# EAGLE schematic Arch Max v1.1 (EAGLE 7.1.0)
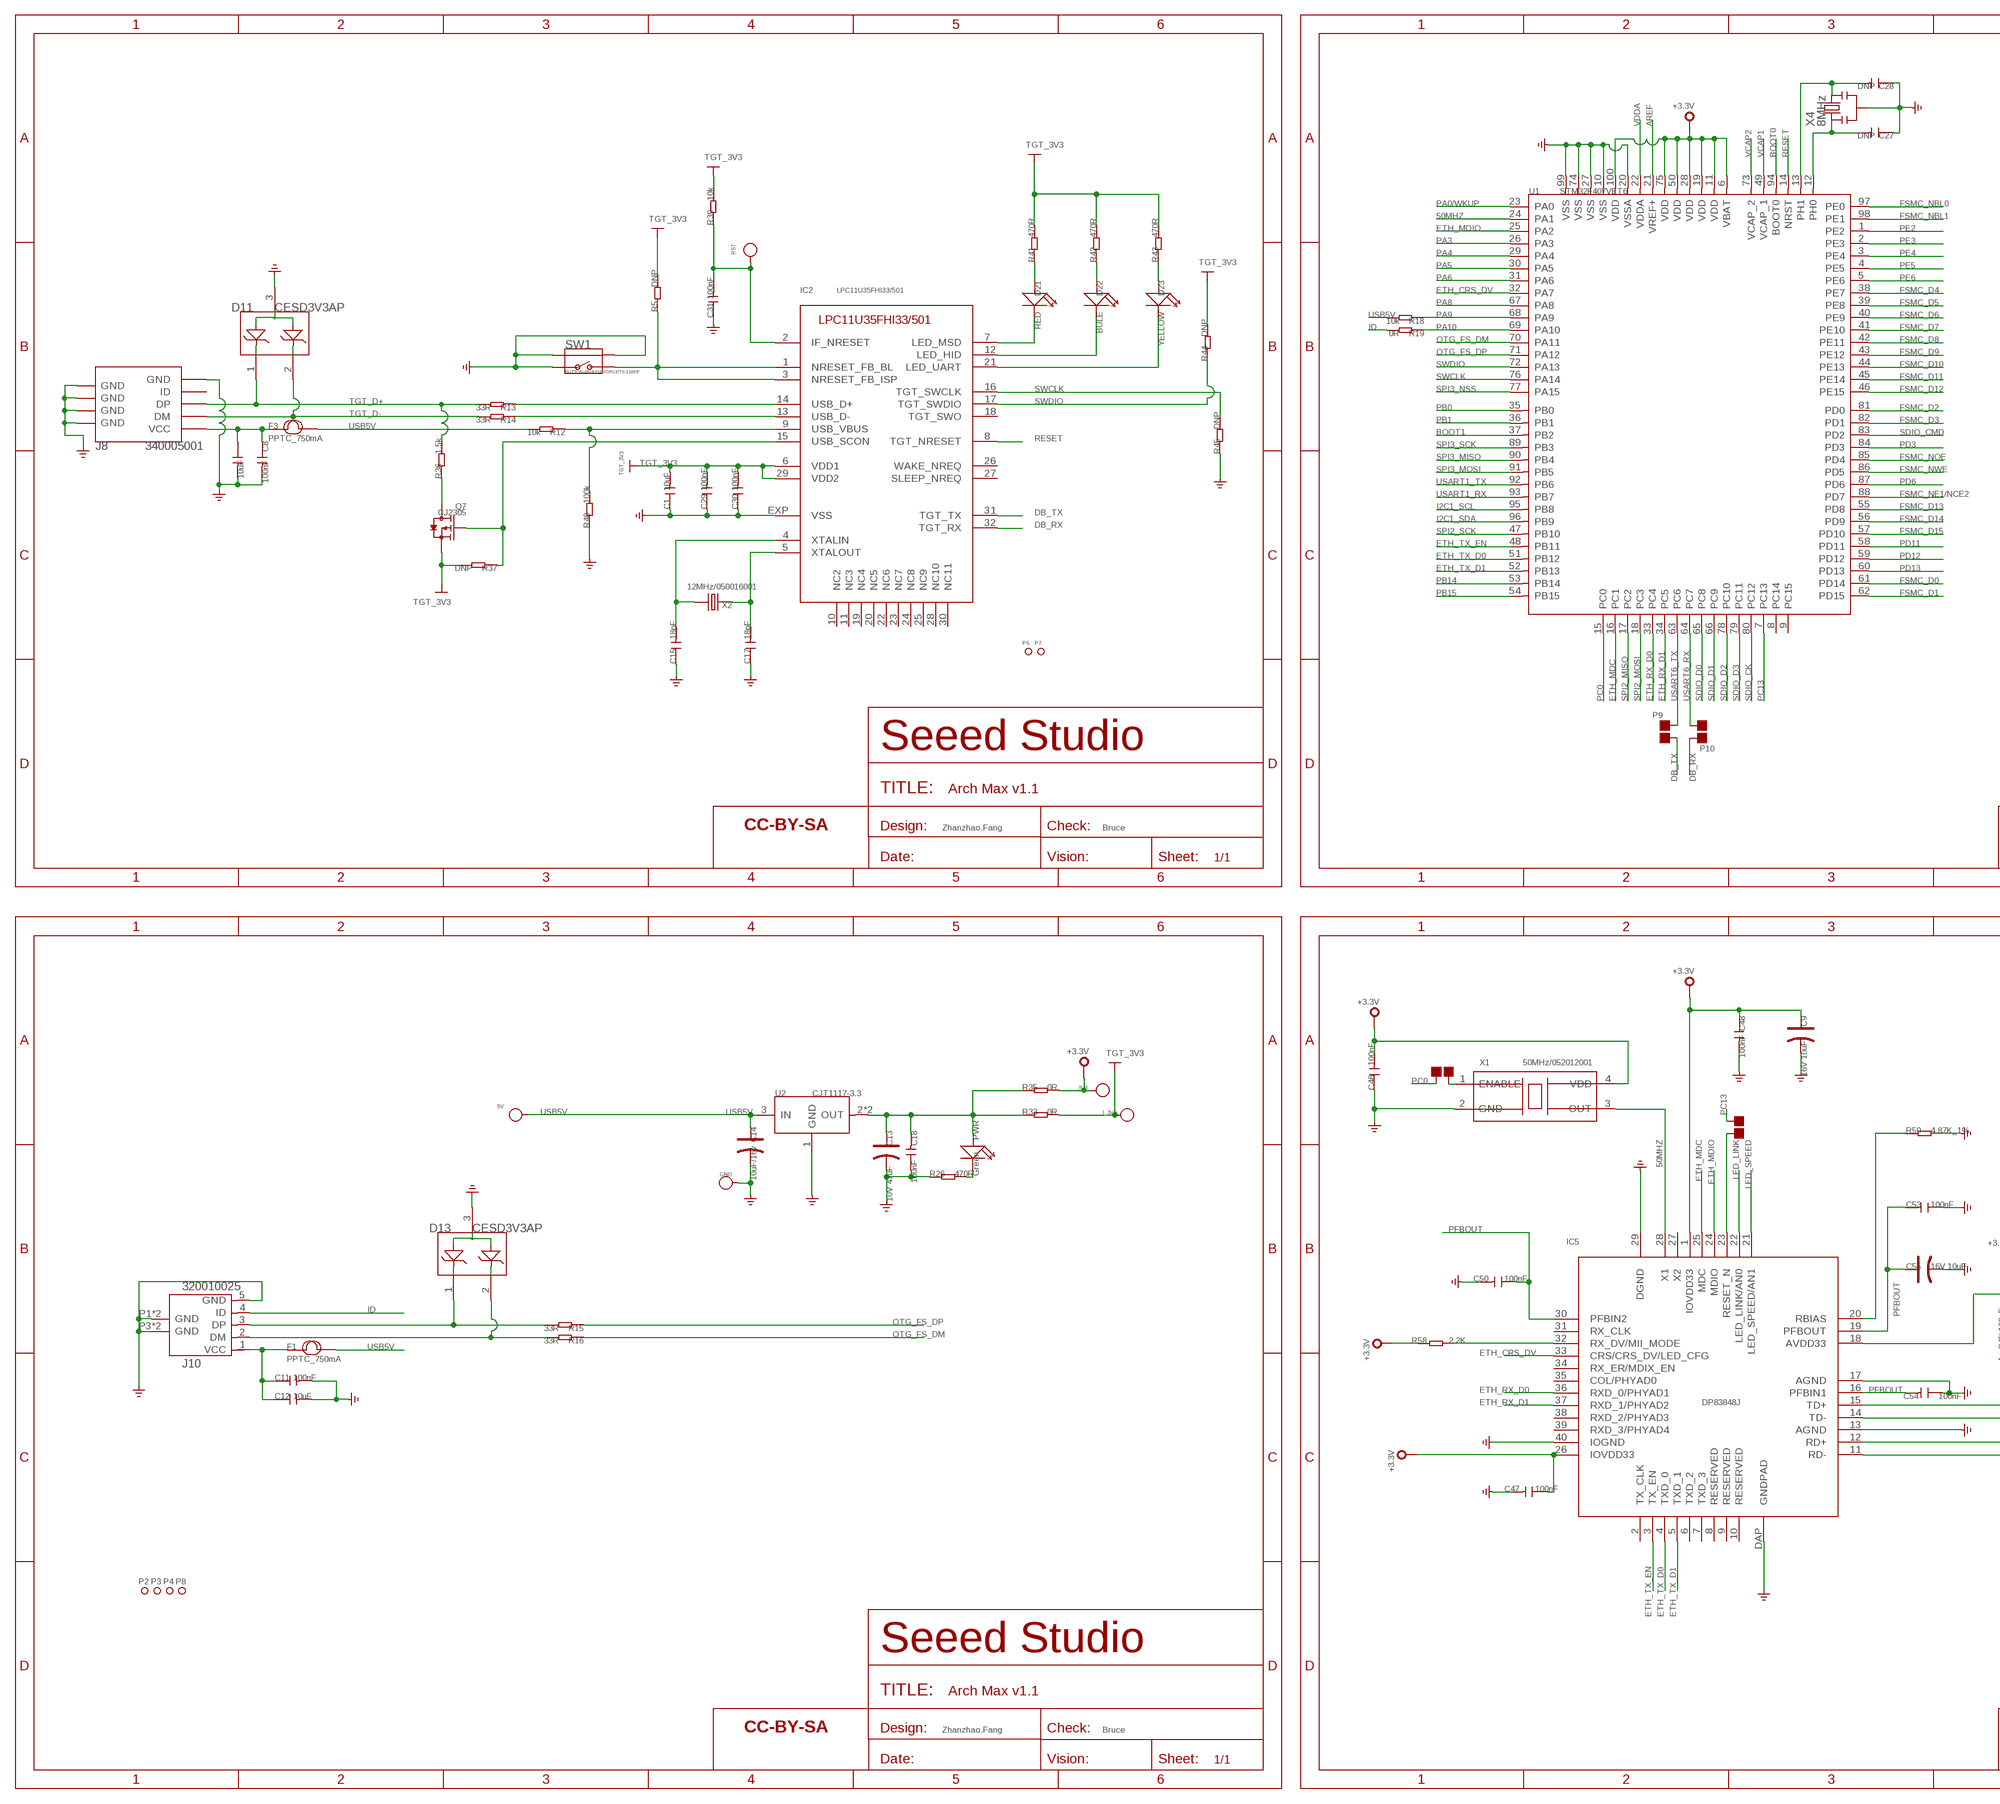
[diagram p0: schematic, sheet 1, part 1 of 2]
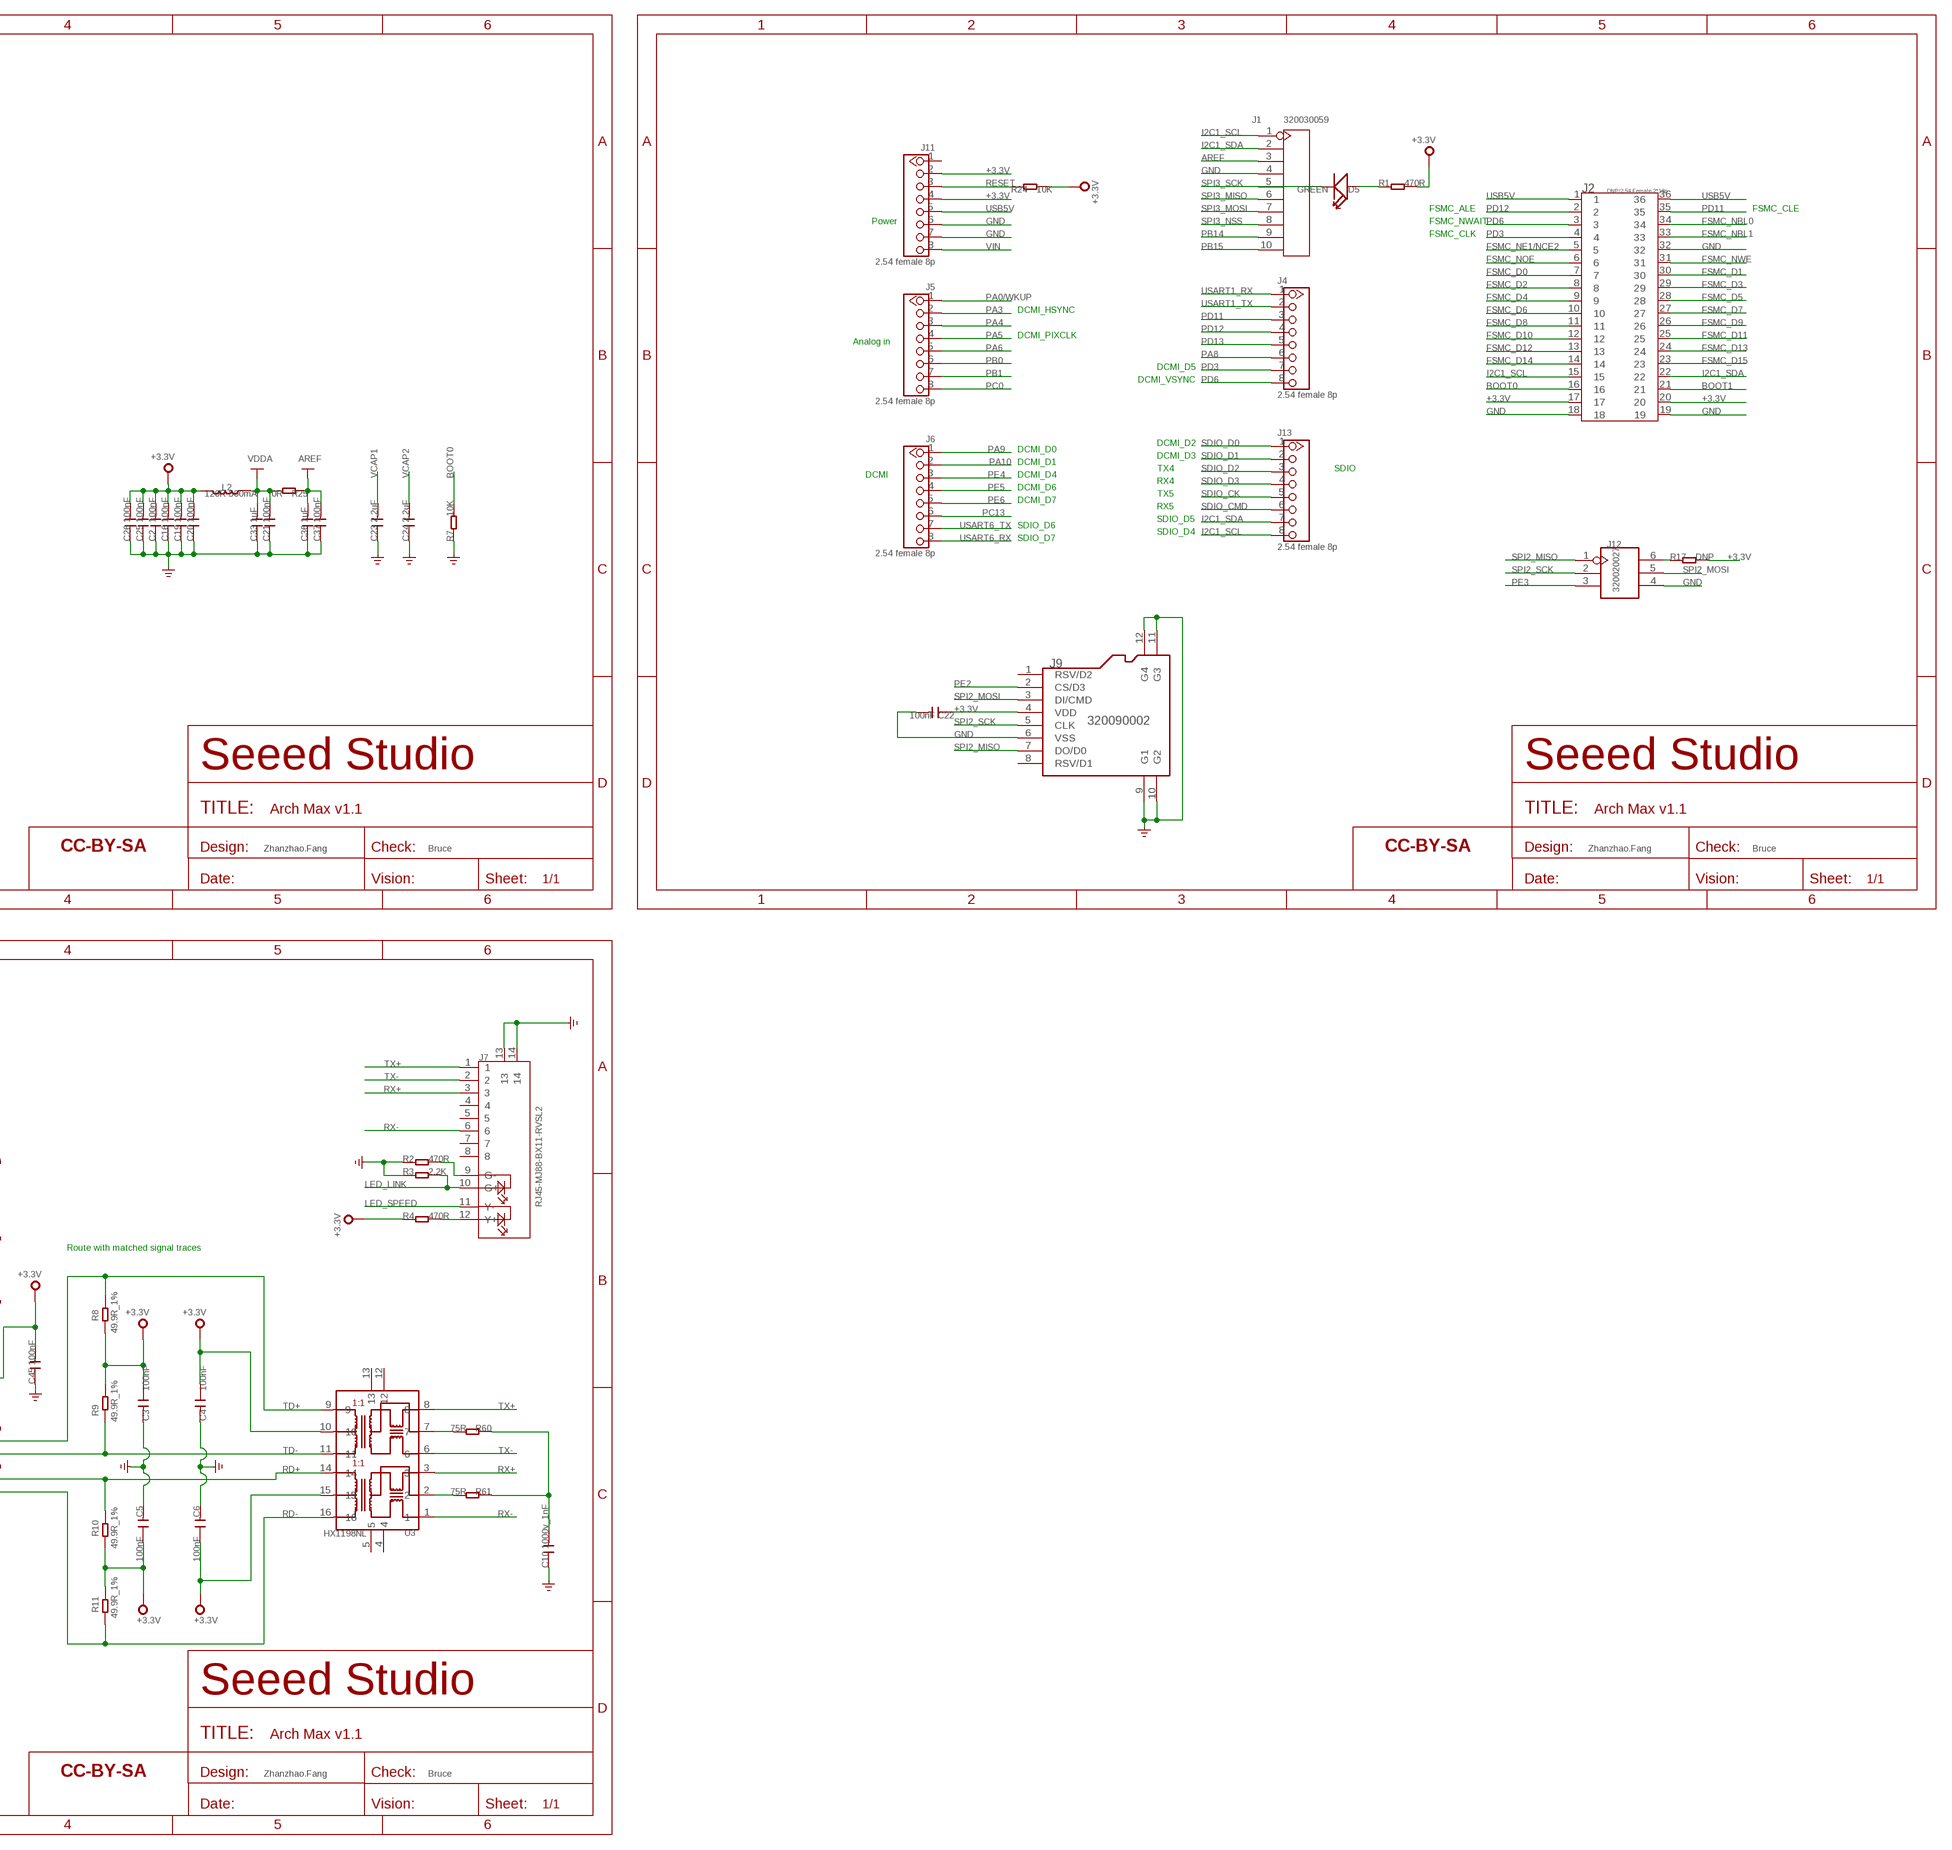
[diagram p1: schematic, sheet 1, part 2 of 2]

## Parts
3V3  NC  PAD-TEST-POINT'4545'  [TP_4545]
5V  NC  PAD-TEST-POINT'4545'  [TP_4545]
C1  10uF  C-0805  [C0805]
C2  100nF  C-0603  [C0603]
C3  100nF  C-0603  [C0603]
C4  100nF  C-0603  [C0603]
C5  100nF  C-0603  [C0603]
C6  100nF  C-0603  [C0603]
C7  10uF  C-0805  [C0805]
C8  100nF  C-0603  [C0603]
C9  16V 10uF  CAP-AVX-A  [AVX-A]
C10  1000v_1nF  C-1206  [C1206]
C11  100nF  C-0603  [C0603]
C12  10uF  C-0805  [C0805]
C13  10V 47uF  CAP-AVX-B  [AVX-B]
C14  10uF/16v  CAP-AVX-A  [AVX-A]
C15  18pF  C-0603  [C0603]
C16  100nF  C-0603  [C0603]
C17  18pF  C-0603  [C0603]
C18  100nF  C-0603  [C0603]
C19  100nF  C-0603  [C0603]
C20  100nF  C-0603  [C0603]
C21  100nF  C-0603  [C0603]
C22  100nF  C-0603  [C0603]
C23  2.2uF  C-0603  [C0603]
C24  2.2uF  C-0603  [C0603]
C25  100nF  C-0603  [C0603]
C26  100nF  C-0603  [C0603]
C27  DNP  C-0603  [C0603]
C28  DNP  C-0603  [C0603]
C29  100nF  C-0603  [C0603]
C30  100nF  C-0603  [C0603]
C31  100nF  C-0603  [C0603]
C33  1uF  C-0603  [C0603]
C36  1uF  C-0603  [C0603]
C37  100nF  C-0603  [C0603]
C45  100nF  C-0603  [C0603]
C46  100nF  C-0603  [C0603]
C47  100nF  C-0603  [C0603]
C48  100nF  C-0603  [C0603]
C50  100nF  C-0603  [C0603]
C53  100nF  C-0603  [C0603]
C54  100nF  C-0603  [C0603]
C55  16V 10uF  CAP-AVX-A  [AVX-A]
D5  GREEN  LED'0603'  [LED-0603]
D11  CESD3V3AP  D-ESD-3P  [SOT23]
D13  CESD3V3AP  D-ESD-3P  [SOT23]
D21  RED  LED'0603'  [LED-0603]
D22  BULE  LED'0603'  [LED-0603]
D23  YELLOW  LED'0603'  [LED-0603]
F1  PPTC_750mA  FUSE'1206'  [F1206]
F3  PPTC_750mA  FUSE'1206'  [F1206]
GND  NC  PAD-TEST-POINT'4545'  [TP_4545]
I_3V3  NC  PAD-TEST-POINT'4545'  [TP_4545]
IC2  LPC11U35FHI33/501  MBED-ICS_IF-LPC11U35  [MBED-ICS_HVQFN33]
IC5  DP83848J  [LLP-40]
J1  320030059  HEADER-10P-2.54  [10P-2.54-65/35MIL]
J2  DNP/2.54 Female 2*18p  HEADER-2X18P  [2.54-2X18P]
J4  2.54 female 8p  HEADER-8P2.54  [CK_1X8]
J5  2.54 female 8p  HEADER-8P2.54  [CK_1X8]
J6  2.54 female 8p  HEADER-8P2.54  [CK_1X8]
J7  RJ45-MJ88-BX11-RVSL2  [RJ45-MJ88-BX11-RVSL2]
J8  340005001  USB-MINIUSB-5P-MICRO  [MICRO-USB]
J9  320090002  HOLDER-MICROSD-8P  [8P-SMD]
J10  320010025  USB-MICRO-5P'AB'  [MICRO-USB-5P-AB]
J11  2.54 female 8p  HEADER-8P2.54  [CK_1X8]
J12  320020027  HEADER-2X3P-65/35MIL  [2X3P-2.54-65/35MIL]
J13  2.54 female 8p  HEADER-8P2.54  [CK_1X8]
L2  120R-500mA  L'0603'  [L0603]
P1  NC  PAD-JUMPER-2P  [2P-SMD-1.78X1.27]
P2  NC  PAD-MARK'ANNULAR'  [ROUND-MARK-1.0]
P3  NC  PAD-MARK'ANNULAR'  [ROUND-MARK-1.0]
P4  NC  PAD-MARK'ANNULAR'  [ROUND-MARK-1.0]
P5  NC  PAD-JUMPER-2P  [2P-SMD-1.78X1.27]
P6  NC  PAD-MARK'ANNULAR'  [ROUND-MARK-1.0]
P7  NC  PAD-MARK'ANNULAR'  [ROUND-MARK-1.0]
P8  NC  PAD-MARK'ANNULAR'  [ROUND-MARK-1.0]
P9  NC  PAD-JUMPER-2P  [2P-SMD-1.78X1.27]
P10  NC  PAD-JUMPER-2P  [2P-SMD-1.78X1.27]
PWR  Green  LED'0603'  [LED-0603]
Q7  CJ2305  MOSFET-P'SI2323CDS/SI2305DS<BR>'  [SOT23]
R1  470R  R-0603  [R0603]
R2  470R  R-0603  [R0603]
R3  2.2K  R-0603  [R0603]
R4  470R  R-0603  [R0603]
R5  DNP  R-0603  [R0603]
R7  10K  R-0603  [R0603]
R8  49.9R_1%  R-0603  [R0603]
R9  49.9R_1%  R-0603  [R0603]
R10  49.9R_1%  R-0603  [R0603]
R11  49.9R_1%  R-0603  [R0603]
R12  10k  R-0603  [R0603]
R13  33R  R-0603  [R0603]
R14  33R  R-0603  [R0603]
R15  33R  R-0603  [R0603]
R16  33R  R-0603  [R0603]
R17  DNP  R-0603  [R0603]
R18  10k  R-0603  [R0603]
R19  0R  R-0603  [R0603]
R24  10K  R-0603  [R0603]
R25  0R  R-0603  [R0603]
R26  470R  R-0603  [R0603]
R33  0R  R-0603  [R0603]
R35  0R  R-0603  [R0603]
R36  1.5k  R-0603  [R0603]
R37  DNP  R-0603  [R0603]
R39  10k  R-0603  [R0603]
R40  100k  R-0603  [R0603]
R41  470R  R-0603  [R0603]
R42  470R  R-0603  [R0603]
R43  470R  R-0603  [R0603]
R44  DNP  R-0603  [R0603]
R45  DNP  R-0603  [R0603]
R58  2.2K  R-0603  [R0603]
R59  4.87K_1%  R-0603  [R0603]
R60  75R  R-0603  [R0603]
R61  75R  R-0603  [R0603]
RST  NC  PAD-TEST-POINT'4545'  [TP_4545]
SW1  BUTTON-4P-REINFORCE'TS-1188E'  [4P-SMD-7X3.5X3.5H]
U1  STM32F407VET6  [LQFP100]
U2  CJT1117-3.3  LD1117S  [SOT-223]
U3  HX1198NL  [SOIC16-9.53]
U$1  SEEEDSTUDIO-OPEN-SCH-FRAME  [SEEEDSTUDIO-PCB-FRAME]
U$2  SEEEDSTUDIO-OPEN-SCH-FRAME  [SEEEDSTUDIO-PCB-FRAME]
U$3  SEEEDSTUDIO-OPEN-SCH-FRAME  [SEEEDSTUDIO-PCB-FRAME]
U$4  SEEEDSTUDIO-OPEN-SCH-FRAME  [SEEEDSTUDIO-PCB-FRAME]
U$5  SEEEDSTUDIO-OPEN-SCH-FRAME  [SEEEDSTUDIO-PCB-FRAME]
X1  50MHz/052012001  CRYSTAL-SPXO  [4P-SMD-5X3.2]
X2  12MHz/050016001  CRYSTAL'5032'  [2P-SMD-5X3.2]
X4  8MHz  CRYSTAL-RESONATOR'SMD'  [3P-SMD-3.6X1.3]

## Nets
50MHZ: IC5.28(X1) U1.24(PA1) X1.3(OUT)
+3.3V: 3V3.T C2.2 C3.1 C4.1 C5.1 C6.1 C9.+ C16.2 C19.2 C20.2 C22.1 C25.2 C26.2 C45.2 C46.2 C47.1 C48.1 IC5.1(IOVDD33) IC5.18(AVDD33) IC5.26(IOVDD33) J2.17 J2.20 J9.4(VDD) J11.2 J11.4 L2.2 R1.2 R4.1 R8.1 R9.2 R10.1 R11.2 R17.2 R24.2 R35.1 R58.1 U1.6(VBAT) U1.11(VDD) U1.19(VDD) U1.28(VDD) U1.50(VDD) U1.75(VDD) U1.100(VDD) U3.10 U3.15 X1.4(VDD)
AREF: C36.2 C37.2 J1.3 R25.1 U1.21(VREF+)
BOOT0: J2.16 R7.2 U1.94(BOOT0)
BOOT1: J2.21 U1.37(PB2)
DB_RX: IC2.32(TGT_RX) P10.2
DB_TX: IC2.31(TGT_TX) P9.1
ETH_CRS_DV: IC5.33(CRS/CRS_DV/LED_CFG) U1.32(PA7)
ETH_MDC: IC5.25(MDC) U1.16(PC1)
ETH_MDIO: IC5.24(MDIO) U1.25(PA2)
ETH_RX_D0: IC5.36(RXD_0/PHYAD1) U1.33(PC4)
ETH_RX_D1: IC5.37(RXD_1/PHYAD2) U1.34(PC5)
ETH_TX_D0: IC5.4(TXD_0) U1.51(PB12)
ETH_TX_D1: IC5.5(TXD_1) U1.52(PB13)
ETH_TX_EN: IC5.3(TX_EN) U1.48(PB11)
FSMC_D0: J2.7 U1.61(PD14)
FSMC_D1: J2.30 U1.62(PD15)
FSMC_D2: J2.8 U1.81(PD0)
FSMC_D3: J2.29 U1.82(PD1)
FSMC_D4: J2.9 U1.38(PE7)
FSMC_D5: J2.28 U1.39(PE8)
FSMC_D6: J2.10 U1.40(PE9)
FSMC_D7: J2.27 U1.41(PE10)
FSMC_D8: J2.11 U1.42(PE11)
FSMC_D9: J2.26 U1.43(PE12)
FSMC_D10: J2.12 U1.44(PE13)
FSMC_D11: J2.25 U1.45(PE14)
FSMC_D12: J2.13 U1.46(PE15)
FSMC_D13: J2.24 U1.55(PD8)
FSMC_D14: J2.14 U1.56(PD9)
FSMC_D15: J2.23 U1.57(PD10)
FSMC_NBL0: J2.34 U1.97(PE0)
FSMC_NBL1: J2.33 U1.98(PE1)
FSMC_NE1/NCE2: J2.5 U1.88(PD7)
FSMC_NOE: J2.6 U1.85(PD4)
FSMC_NWE: J2.31 U1.86(PD5)
GND: C1.1 C2.1 C3.2 C4.2 C5.2 C6.2 C7.2 C8.2 C9.- C10.1 C11.2 C12.2 C13.- C14.- C15.1 C16.1 C17.1 C18.1 C19.1 C20.1 C21.1 C22.2 C23.1 C24.1 C25.1 C26.1 C27.1 C28.1 C29.1 C30.1 C31.1 C33.1 C36.1 C37.1 C45.1 C46.1 C47.2 C48.2 C50.2 C53.1 C54.1 C55.- D11.3 D13.3 GND.T IC2.EXP(VSS) IC5.13(AGND) IC5.17(AGND) IC5.29(DGND) IC5.40(IOGND) IC5.DAP(GNDPAD) J1.4 J2.18 J2.19 J2.32 J7.13 J7.14 J8.5(GND) J8.S1(GND) J8.S2(GND) J8.S3(GND) J8.S4(GND) J8.S5(GND) J8.S6(GND) J9.6(VSS) J9.9(G1) J9.10(G2) J9.11(G3) J9.12(G4) J10.5(GND) J10.P1(GND) J10.P2(GND) J10.P3(GND) J10.P4(GND) J11.6 J11.7 J12.4 R2.1 R3.1 R7.1 R26.1 R40.1 R45.1 R59.2 SW1.1 SW1.S1 SW1.S2 U1.10(VSS) U1.20(VSSA) U1.27(VSS) U1.74(VSS) U1.99(VSS) U2.1(GND) X1.2(GND) X4.2
GREEN: D22.- IC2.12(LED_HID)
GREEN1: D21.- IC2.7(LED_MSD)
I2C1_SCL: J1.1 J2.15 J13.8 U1.95(PB8)
I2C1_SDA: J1.2 J2.22 J13.7 U1.96(PB9)
ID: J10.4(ID) R19.2
LED_LINK: IC5.22(LED_LINK/AN0) J7.10(G+) R3.2
LED_SPEED: IC5.21(LED_SPEED/AN1) J7.11(Y-)
N$1: C11.1 C12.1 F1.1 J10.1(VCC)
N$2: J12.6 R17.1
N$3: IC2.1(NRESET_FB_BL) IC2.3(NRESET_FB_ISP) R5.1 SW1.2
N$4: IC5.23(RESET_N) P1.2
N$5: IC2.9(USB_VBUS) R12.1 R40.2
N$6: J7.9(G-) R2.2
N$7: J7.12(Y+) R4.2
N$8: D5.+ R1.1
N$9: P5.2 X1.1(ENABLE)
N$10: C7.1 C8.1 F3.1 J8.1(VCC)
N$12: IC2.14(USB_D+) R13.1
N$13: IC2.13(USB_D-) R14.1
N$15: D13.1 J10.3(DP) R15.2
N$18: PWR.- R26.2
N$22: D13.2 J10.2(DM) R16.2
N$23: C13.+ C18.2 PWR.+ R33.1 R35.2 U2.2(OUT) U2.TER(OUT)
N$24: C31.2 IC2.2(IF_NRESET) R39.1 RST.T
N$25: IC2.15(USB_SCON) Q7.1(G) R37.1
N$26: D22.+ R42.1
N$27: Q7.3(D) R36.1
N$28: D21.+ R41.1
N$32: D23.- IC2.21(LED_UART)
N$33: D23.+ R43.1
N$34: C15.2 IC2.4(XTALIN) X2.2
N$37: C17.2 IC2.5(XTALOUT) X2.1
N$56: R61.2 U3.2
N$58: R60.2 U3.7
N$59: C10.2 R60.1 R61.1
N$123: IC5.20(RBIAS) R59.1
N$127: IC5.32(RX_DV/MII_MODE) R58.2
OTG_FS_DM: R16.1 U1.70(PA11)
OTG_FS_DP: R15.1 U1.71(PA12)
PA0/WKUP: J5.1 U1.23(PA0)
PA3: J5.2 U1.26(PA3)
PA4: J5.3 U1.29(PA4)
PA5: J5.4 U1.30(PA5)
PA6: J5.5 U1.31(PA6)
PA8: J4.6 U1.67(PA8)
PA9: J6.1 R18.1 U1.68(PA9)
PA10: J6.2 R19.1 U1.69(PA10)
PB0: J5.6 U1.35(PB0)
PB1: J5.7 U1.36(PB1)
PB14: J1.9 U1.53(PB14)
PB15: J1.10 U1.54(PB15)
PC0: J5.8 P5.1 U1.15(PC0)
PC13: J6.6 P1.1 U1.7(PC13)
PD3: J2.4 J4.7 U1.84(PD3)
PD6: J2.3 J4.8 U1.87(PD6)
PD11: J2.35 J4.3 U1.58(PD11)
PD12: J2.2 J4.4 U1.59(PD12)
PD13: J4.5 U1.60(PD13)
PE2: J9.2(CS/D3) U1.1(PE2)
PE3: J12.3 U1.2(PE3)
PE4: J6.3 U1.3(PE4)
PE5: J6.4 U1.4(PE5)
PE6: J6.5 U1.5(PE6)
PFBOUT: C50.1 C53.2 C54.2 C55.+ IC5.16(PFBIN1) IC5.19(PFBOUT) IC5.30(PFBIN2)
RD+: IC5.12(RD+) R10.2 U3.14
RD-: IC5.11(RD-) R11.1 U3.16
RESET: IC2.8(TGT_NRESET) J11.3 R24.1 U1.14(NRST)
RX+: J7.3 U3.3
RX-: J7.6 U3.1
SDIO_CK: J13.5 U1.80(PC12)
SDIO_CMD: J13.6 U1.83(PD2)
SDIO_D0: J13.1 U1.65(PC8)
SDIO_D1: J13.2 U1.66(PC9)
SDIO_D2: J13.3 U1.78(PC10)
SDIO_D3: J13.4 U1.79(PC11)
SPI2_MISO: J9.7(DO/D0) J12.1 U1.17(PC2)
SPI2_MOSI: J9.3(DI/CMD) J12.5 U1.18(PC3)
SPI2_SCK: J9.5(CLK) J12.2 U1.47(PB10)
SPI3_MISO: J1.6 U1.90(PB4)
SPI3_MOSI: J1.7 U1.91(PB5)
SPI3_NSS: J1.8 U1.77(PA15)
SPI3_SCK: D5.- J1.5 U1.89(PB3)
SWCLK: IC2.16(TGT_SWCLK) R45.2 U1.76(PA14)
SWDIO: IC2.17(TGT_SWDIO) R44.1 U1.72(PA13)
TD+: IC5.15(TD+) R8.2 U3.9
TD-: IC5.14(TD-) R9.1 U3.11
TGT_3V3: C1.2 C29.2 C30.2 I_3V3.T IC2.6(VDD1) IC2.29(VDD2) Q7.2(S) R5.2 R33.2 R37.2 R39.2 R41.2 R42.2 R43.2 R44.2
TGT_D+: D11.1 J8.3(DP) R13.2 R36.2
TGT_D-: D11.2 J8.2(DM) R14.2
TX+: J7.1 U3.8
TX-: J7.2 U3.6
USART1_RX: J4.1 U1.93(PB7)
USART1_TX: J4.2 U1.92(PB6)
USART6_RX: J6.8 P10.1 U1.64(PC7)
USART6_TX: J6.7 P9.2 U1.63(PC6)
USB5V: 5V.T C14.+ F1.2 F3.2 J2.1 J2.36 J11.5 R12.2 R18.2 U2.3(IN)
VCAP1: C23.2 U1.49(VCAP_1)
VCAP2: C24.2 U1.73(VCAP_2)
VDDA: C21.2 C33.2 L2.1 R25.2 U1.22(VDDA)
VIN: J11.8
XTALIN: C27.2 U1.12(PH0) X4.1
XTALOUT: C28.2 U1.13(PH1) X4.3
Unconnected: IC2.10(NC2) IC2.11(NC3) IC2.18(TGT_SWO) IC2.19(NC4) IC2.20(NC5) IC2.22(NC6) IC2.23(NC7) IC2.24(NC8) IC2.25(NC9) IC2.26(WAKE_NREQ) IC2.27(SLEEP_NREQ) IC2.28(NC10) IC2.30(NC11) IC5.2(TX_CLK) IC5.6(TXD_2) IC5.7(TXD_3) IC5.8(RESERVED) IC5.9(RESERVED) IC5.10(RESERVED) IC5.27(X2) IC5.31(RX_CLK) IC5.34(RX_ER/MDIX_EN) IC5.35(COL/PHYAD0) IC5.38(RXD_2/PHYAD3) IC5.39(RXD_3/PHYAD4) J7.4 J7.5 J7.7 J7.8 J8.4(ID) J9.1(RSV/D2) J9.8(RSV/D1) J11.1 U1.8(PC14) U1.9(PC15) U3.4 U3.5 U3.12 U3.13

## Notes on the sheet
- FSMC_ALE | FSMC_CLE
- Power | FSMC_NWAIT
- FSMC_CLK
- DCMI_HSYNC
- DCMI_PIXCLK
- Analog in
- DCMI_D5
- DCMI_VSYNC
- DCMI_D2
- DCMI_D0
- DCMI_D3
- DCMI_D1
- TX4 | SDIO
- DCMI | DCMI_D4
- RX4
- DCMI_D6
- TX5
- DCMI_D7
- RX5
- SDIO_D5
- SDIO_D6
- SDIO_D4
- SDIO_D7
- Zhanzhao.Fang | Bruce | Zhanzhao.Fang | Bruce | Zhanzhao.Fang | Bruce
- Route with matched signal traces
- Zhanzhao.Fang | Bruce | Zhanzhao.Fang | Bruce

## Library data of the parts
3V3 5V GND I_3V3 RST = Discrete:PAD-TEST-POINT; PARTNO: DNP
C1-C8 C10-C12 C15-C31 C33 C36 C37 C45-C48 C50 C53 C54 = Discrete:C*: Ceramic Capacitors
C9 C13 C14 C55 = Discrete:CAP*: Electrolytic Capacitors,Tantalum Capacitors and Super Capacitors
D5 D21-D23 PWR = Discrete:LED*
D11 D13 = Discrete:D-ESD-3P
F1 F3 = Discrete:FUSE
IC2 = Arch_M4:MBED-ICS_IF-LPC11U35
IC5 = mbed:DP83848J: National Semiconductor DP83848J PHYTER Mini LS Single Port 10/100 Ethernet Transceiver
J1 = Connector-new:HEADER-10P
J2 = Connector:HEADER-2X18P
J4-J6 J11 J13 = Connector:HEADER-8P
J7 = Connector:RJ45-MJ88-BX11-RVSL2: Modular Jack 8P8C,R/A,With LED
J8 = Connector :USB-MINIUSB-5P
J9 = Connector :HOLDER-MICROSD-8P
J10 = template :USB-MICRO-5P: ST-USB-001L5 The Size of ST-USB-001L5 is 8.0X2.35X5.61mm.when you use it ,you need know that the Size of pin is only 1.6MM.
J12 = Connector :HEADER-2X3P
L2 = Discrete:L*
P1 P5 P9 P10 = Discrete:PAD-JUMPER-2P; PARTNO: DNP
P2-P4 P8 = Discrete-new:PAD-MARK; PARTNO: DNP
P6 P7 = Discrete:PAD-MARK; PARTNO: DNP
Q7 = Discrete:MOSFET-P
R1-R5 R7-R19 R24-R26 R33 R35-R37 R39-R45 R58-R61 = Discrete:R*
SW1 = Discrete:BUTTON-4P-REINFORCE: TS-1188E http://www.best-dz.com/?thread-374-2.html
U1 = template :STM32F407VET6: ARM Cortex-M4 32b MCU+FPU,210 DMIPS,up to 1MB Flash/192+4KB RAM,USB OTG HS/FS, Ethernet ,17TIMs,3ADCs,15comm.interfaces&camera
U2 = IC:LD1117: Low Drop Fixed And Adjustable Positive Voltage Regulators http://www.datasheetcatalog.org/datasheet/SGSThomsonMicroelectronics/mXuqtqv.pdf
U3 = IC:HX1198NL: 10/100BASE-T Single Port Surface Mount Magnetics With Various Turns Ratios
U$1-U$5 = moudle-new:SEEEDSTUDIO-OPEN-SCH-FRAME
X1 = Discrete:CRYSTAL-SPXO
X2 = Discrete:CRYSTAL*: CRYSTAL
X4 = Discrete:CRYSTAL-RESONATOR: Resonator Small SMD resonator. This is the itty bitty 10/20MHz resonators with built in caps. CSTCE10M0G55 and CSTCE20M0V53. Footprint has been reviewed closely but hasn't been tested yet.

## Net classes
0 default: width 0.102 mm, drill 0.203 mm, clearance 0.102 mm

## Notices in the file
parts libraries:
moudle-new: This work is licensed under the Creative Commons Attribution 4.0 International License.
To view a copy of this license,visit:
http://creativecommons.org/licenses/by-sa/4.0
moudle-new: CC-BY-SA
